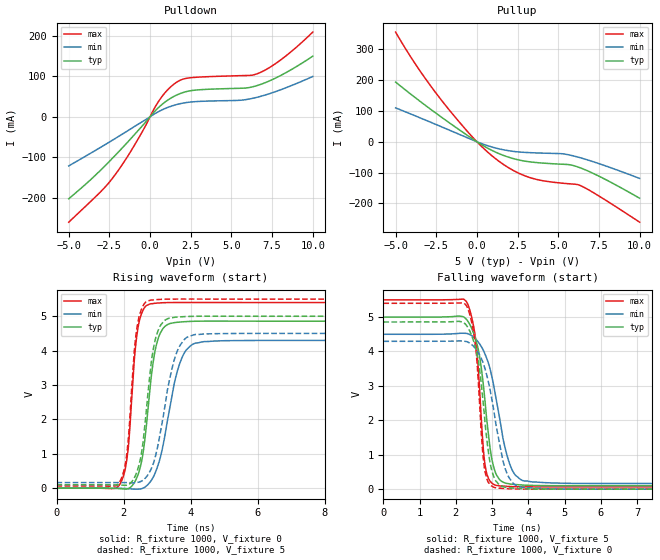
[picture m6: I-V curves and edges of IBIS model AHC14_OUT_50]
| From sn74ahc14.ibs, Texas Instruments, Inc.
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[Model]   AHC14_OUT_50
Model_type  Output
Vref =   0
Rref =   1000
Cref =   50p
Vmeas =   2.5
| variable   typ   min   max
C_comp   2.62pF   1.48pF   3.65pF
| C_pullup   2.77pF   1.48pF   3.65pF
| C_pulldown   2.46pF   1.58pF   3.39pF
[Temperature Range]   40   100   -40
| Ambient temperature   25   85   -40
[Voltage range]   5   4.5   5.5
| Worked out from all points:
|   slope of the pulldown table from 0 to 0.75 V, typ, clamps not added: 24.2 ohm
|   slope of the pullup table from 0 to 0.75 V, typ, clamps not added: 32.1 ohm
|   rising waveform, R_fixture 1000, V_fixture 0: 20-80 % time 346ps typ, 527ps min, 251ps max; typ from 0 V to 4.86 V
|   falling waveform, R_fixture 1000, V_fixture 5: 20-80 % time 333ps typ, 492ps min, 221ps max; typ from 5 V to 0.101 V
|   rising waveform, R_fixture 1000, V_fixture 5: 20-80 % time 339ps typ, 509ps min, 251ps max; typ from 0.101 V to 5 V
|   falling waveform, R_fixture 1000, V_fixture 0: 20-80 % time 322ps typ, 472ps min, 219ps max; typ from 4.86 V to 0 V
[Pulldown]
| AHC14_OUT_50
|   Voltage   I(typ)   I(min)   I(max)
-5V       -203.2mA   -121.7mA   -261.1mA
-3.07V    -133.5mA   -76.46mA   -187mA
-2.27V    -101mA     -57.05mA   -150.2mA
-1.02V    -46.97mA   -25.75mA   -74.62mA
510mV     22.36mA    12.39mA    37.2mA
970mV     37.83mA    21.14mA    61.73mA
1.46V     50.19mA    28.2mA     80.49mA
2.405V    63.82mA    36.03mA    96.15mA
5.545V    70.46mA    40.77mA    101.7mA
6.605V    77.49mA    48.42mA    106.7mA
8.09V     103.5mA    67.7mA     142.5mA
10V       149.9mA    99.56mA    209.6mA
[Pullup]
| AHC14_OUT_50
|   Voltage   I(typ)   I(min)   I(max)
-5V       193.4mA    109.9mA    355.5mA
-3.6V     135.3mA    79.82mA    237.4mA
-2.035V   74.16mA    45.29mA    124.9mA
-215mV    7.5mA      4.696mA    11.93mA
1.165V    -34.04mA   -20.45mA   -55.72mA
2.21V     -54.21mA   -30.99mA   -92.25mA
3.26V     -65.13mA   -35.31mA   -116.2mA
4.09V     -69.26mA   -36.91mA   -126.6mA
5.215V    -72.73mA   -38.72mA   -134.1mA
6.085V    -79.6mA    -47.92mA   -137.9mA
7.11V     -101.6mA   -64.04mA   -163.3mA
10V       -183mA     -118.8mA   -260.7mA
[Ramp]
| AHC14_OUT_50
| variable   typ   min   max
dV/dt_r   2.93/3.54E-10   2.59/5.50E-10   3.25/2.59E-10
dV/dt_f   2.96/3.41E-10   2.62/5.12E-10   3.28/2.25E-10
R_load = 1000
[Rising Waveform]
| AHC14_OUT_50
R_fixture =   1000
C_fixture =   0
L_fixture =   0
V_fixture =   0
V_fixture_min = 0
V_fixture_max = 0
|   Time   V(typ)   V(min)   V(max)
0s        1.078nV    1.79nV     663.1pV
1.91ns    -13.16mV   -3.341mV   149.2mV
2.135ns   -12.52mV   -11.88mV   1.116V
2.32ns    159.1mV    -26.57mV   3.712V
2.45ns    449mV      -25.77mV   4.768V
2.6ns     1.144V     11.09mV    5.212V
2.96ns    4.086V     482.8mV    5.38V
3.695ns   4.833V     3.677V     5.401V
4.41ns    4.859V     4.264V     5.401V
50ns      4.857V     4.295V     5.4V
[Falling Waveform]
| AHC14_OUT_50
R_fixture =   1000
C_fixture =   0
L_fixture =   0
V_fixture =   5
V_fixture_min = 4.5
V_fixture_max = 5.5
|   Time   V(typ)   V(min)   V(max)
0s        5V         4.5V       5.5V
2.305ns   4.917V     4.524V     5.428V
2.555ns   4.325V     4.354V     4.291V
2.755ns   3.067V     4.041V     1.218V
2.83ns    2.275V     3.861V     560.2mV
3ns       843.1mV    3.24V      169.2mV
3.215ns   268.6mV    2.021V     93.52mV
3.635ns   136.5mV    417.2mV    70.26mV
4.645ns   100.9mV    179.5mV    65.17mV
50ns      100.8mV    165mV      65.08mV
[Rising Waveform]
| AHC14_OUT_50
R_fixture =   1000
C_fixture =   0
L_fixture =   0
V_fixture =   5
V_fixture_min = 4.5
V_fixture_max = 5.5
|   Time   V(typ)   V(min)   V(max)
0s        100.8mV    165mV      65.08mV
1.905ns   91.41mV    164.6mV    222.4mV
2.115ns   94.45mV    163.6mV    1.157V
2.425ns   554.4mV    171.1mV    4.806V
2.575ns   1.291V     229.4mV    5.291V
2.825ns   3.638V     565.3mV    5.472V
3.085ns   4.705V     1.549V     5.491V
3.55ns    4.974V     3.847V     5.5V
4.165ns   5V         4.474V     5.5V
50ns      5V         4.5V       5.5V
[Falling Waveform]
| AHC14_OUT_50
R_fixture =   1000
C_fixture =   0
L_fixture =   0
V_fixture =   0
V_fixture_min = 0
V_fixture_max = 0
|   Time   V(typ)   V(min)   V(max)
0s        4.857V     4.295V     5.4V
2.3ns     4.748V     4.287V     5.318V
2.555ns   4.061V     4.067V     4.049V
2.715ns   2.922V     3.767V     1.436V
2.8ns     2.013V     3.517V     543.8mV
2.96ns    683.9mV    2.804V     115.7mV
3.165ns   163.1mV    1.552V     29.02mV
3.58ns    30.28mV    172mV      6.594mV
4.545ns   704.8uV    11.61mV    378.9uV
50ns      -5.204nV   8.759nV    -5.85nV
